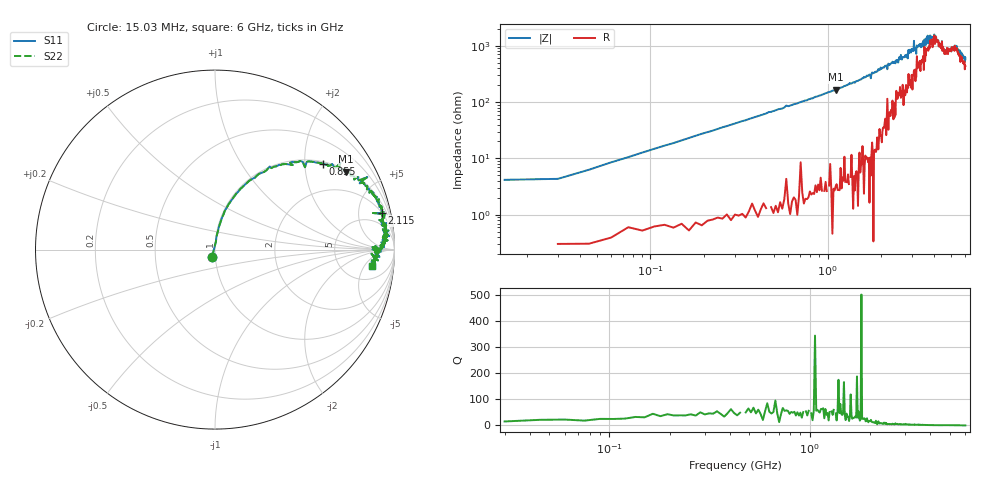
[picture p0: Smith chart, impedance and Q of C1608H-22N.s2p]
!	Network	Analyzer	HP8753E.07.74:	Oct	30	2002	Serial	No.	JP38451487
!	Hewlett-Packard
!	7	Sep	2009	10:21:33
!	Frequency	S11	S21	S12	S22
#	HZ	S	RI	R	50
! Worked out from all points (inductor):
!   400 points, 15.03 MHz to 6 GHz, reference 50 ohm
!   read as one part in series: L = 22.3 nH near 45.03 MHz
!   highest Q = 58.9 at 1.11 GHz (marker M1), where L = 23.9 nH
!   self-resonance near 4.262 GHz
!   S11 on the Smith chart (normalised r, x): 15.03 MHz: 0.97, -0.07; 855 MHz: 1.07, +2.48; 2.115 GHz: 2.01, +8.77; 6 GHz: 10, -8
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1.502992e7  -0.0161 -0.0386  1.02 0.0386  1.02 0.0386  -0.0161 -0.0386
1.050295e8  0.0274 0.143  0.973 -0.143  0.973 -0.143  0.0274 0.143
2.550287e8  0.119 0.312  0.881 -0.312  0.881 -0.312  0.119 0.312
8.550257e8  0.603 0.476  0.397 -0.476  0.397 -0.476  0.603 0.476
1.020025e9  0.689 0.452  0.311 -0.452  0.311 -0.452  0.689 0.452
1.110024e9  0.731 0.434  0.269 -0.434  0.269 -0.434  0.731 0.434
2.01002e9  0.924 0.235  0.0759 -0.235  0.0759 -0.235  0.924 0.235
2.115019e9  0.93 0.204  0.0702 -0.204  0.0702 -0.204  0.93 0.204
3.015015e9  0.967 0.106  0.0329 -0.106  0.0329 -0.106  0.967 0.106
3.075015e9  0.97 0.0742  0.0299 -0.0742  0.0299 -0.0742  0.97 0.0742
3.165014e9  0.935 0.114  0.0647 -0.114  0.0647 -0.114  0.935 0.114
3.195014e9  0.935 0.0667  0.0646 -0.0667  0.0646 -0.0667  0.935 0.0667
3.495013e9  0.953 0.0879  0.0466 -0.0879  0.0466 -0.0879  0.953 0.0879
3.675012e9  0.962 0.0515  0.0382 -0.0515  0.0382 -0.0515  0.962 0.0515
3.91501e9  0.926 0.0404  0.0745 -0.0404  0.0745 -0.0404  0.926 0.0404
4.00501e9  0.942 0.0141  0.058 -0.0141  0.058 -0.0141  0.942 0.0141
4.03501e9  0.921 0.0229  0.0788 -0.0229  0.0788 -0.0229  0.921 0.0229
4.425008e9  0.924 -0.0115  0.0761 0.0115  0.0761 0.0115  0.924 -0.0115
4.455008e9  0.89 0.000854  0.11 -0.000854  0.11 -0.000854  0.89 0.000854
4.575007e9  0.878 0.013  0.122 -0.013  0.122 -0.013  0.878 0.013
5.010005e9  0.897 0.00259  0.103 -0.00259  0.103 -0.00259  0.897 0.00259
6e9  0.875 -0.0888  0.125 0.0888  0.125 0.0888  0.875 -0.0888
